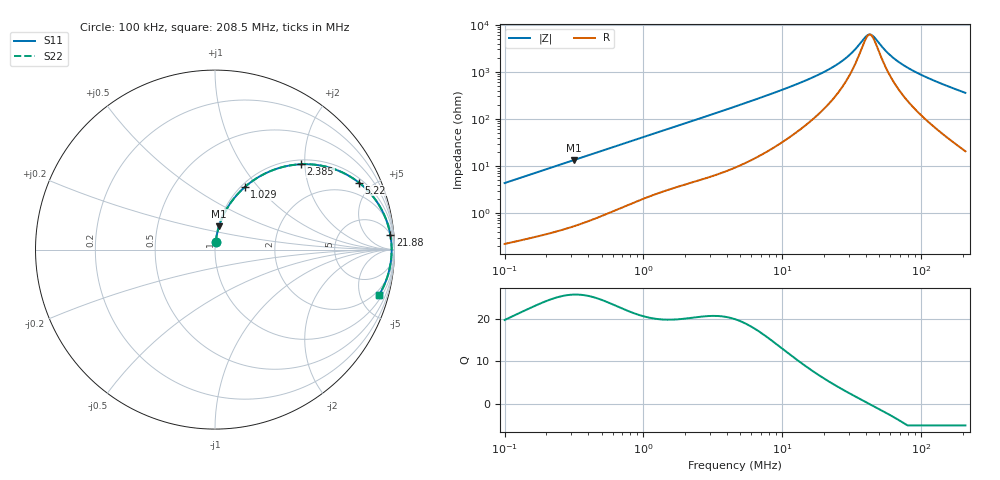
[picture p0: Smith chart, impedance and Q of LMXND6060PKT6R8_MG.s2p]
! LMXND6060PKT6R8_MG  S-PARAMETER MODEL  ( General Type )
! Model Generated by TAIYO YUDEN Corporation (https://www.yuden.co.jp/en/)
! Version 1.0
! TAIYO YUDEN Control No. 191025NI43SB-FBB
! Copyright(c) 2019 TAIYO YUDEN CO.,LTD. All Rights Reserved.
! Product Description (link to TY-COMPAS)
! https://ds.yuden.co.jp/TYCOMPAS/or/detail?pn=LMXND6060PKT6R8MMG&u=M
! Products Name : Inductors
! Characteristics :
!  Inductance : 6.8 uH , SRF(min) : 30 MHz , DC Resistance(max) : 0.138 Ohm
!  Rated Current : Saturation :1700 mA , Temp Rise : 1650 mA (40 degC)
!  Case Size : 6.0 x 6.0 / 0.236 x 0.236 [mm/inch] , Thickness : 1.4 / 0.055 [mm/inch]
!  (Conditions: Temperature = 25 degC , DC Bias Current/Voltage = 0A / 0V)
! External Node Assignments :
!  1  o---GGG---o  2
! GND o---------o GND
! Frequency Range : 0.1MHz  -  208.503118MHz  [ 402 STEP ]
# MHz S RI R 50
! Freq[MHz].  S11 Real  S11 Imag  S21 Real  S21 Imag  S12 Real  S12 Imag  S22 Real  S22 Imag
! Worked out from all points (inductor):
!   401 points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, 100 kHz to 208.5 MHz, reference 50 ohm
!   read as one part in series: L = 6.85 uH near 103.9 kHz
!   highest Q = 25.6 at 314.7 kHz (marker M1), where L = 6.75 uH
!   self-resonance near 42.64 MHz
!   S11 on the Smith chart (normalised r, x): 100 kHz: 1.00, +0.09; 1.029 MHz: 1.04, +0.85; 2.385 MHz: 1.09, +1.92; 5.22 MHz: 1.22, +4.19; 21.88 MHz: 5, +23; 208.5 MHz: 1.41, -7.15
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0.1  0.00405 0.043  0.9959 -0.043  0.9959 -0.043  0.00405 0.043
0.314678  0.0224 0.1298  0.9776 -0.1298  0.9776 -0.1298  0.0224 0.1298
0.359709  0.0282 0.1471  0.9718 -0.1471  0.9718 -0.1471  0.0282 0.1471
0.638094  0.0759 0.2439  0.9241 -0.2439  0.9241 -0.2439  0.0759 0.2439
1.028796  0.1647 0.3472  0.8353 -0.3472  0.8353 -0.3472  0.1647 0.3472
1.293906  0.2305 0.3967  0.7695 -0.3967  0.7695 -0.3967  0.2305 0.3967
2.384689  0.48 0.4756  0.52 -0.4756  0.52 -0.4756  0.48 0.4756
3.237399  0.6212 0.4614  0.3788 -0.4614  0.3788 -0.4614  0.6212 0.4614
4.654297  0.7656 0.3991  0.2344 -0.3991  0.2344 -0.3991  0.7656 0.3991
5.219642  0.8023 0.373  0.1977 -0.373  0.1977 -0.373  0.8023 0.373
8.74341  0.9135 0.2486  0.0865 -0.2486  0.0865 -0.2486  0.9135 0.2486
16.42508  0.9673 0.125  0.0327 -0.125  0.0327 -0.125  0.9673 0.125
21.87632  0.977 0.0821  0.023 -0.0821  0.023 -0.0821  0.977 0.0821
29.6988  0.9823 0.0425  0.0177 -0.0425  0.0177 -0.0425  0.9823 0.0425
39.55538  0.9841 0.00867  0.0159 -0.00867  0.0159 -0.00867  0.9841 0.00867
41.8889  0.9842 0.00206  0.0158 -0.00206  0.0158 -0.00206  0.9842 0.00206
45.21578  0.9842 -0.00675  0.0158 0.00675  0.0158 0.00675  0.9842 -0.00675
59.08252  0.9828 -0.0382  0.0172 0.0382  0.0172 0.0382  0.9828 -0.0382
72.90118  0.9801 -0.0645  0.0199 0.0645  0.0199 0.0645  0.9801 -0.0645
95.25845  0.9737 -0.1018  0.0263 0.1018  0.0263 0.1018  0.9737 -0.1018
139.5916  0.9555 -0.166  0.0445 0.166  0.0445 0.166  0.9555 -0.166
208.5031  0.9154 -0.2511  0.0846 0.2511  0.0846 0.2511  0.9154 -0.2511
